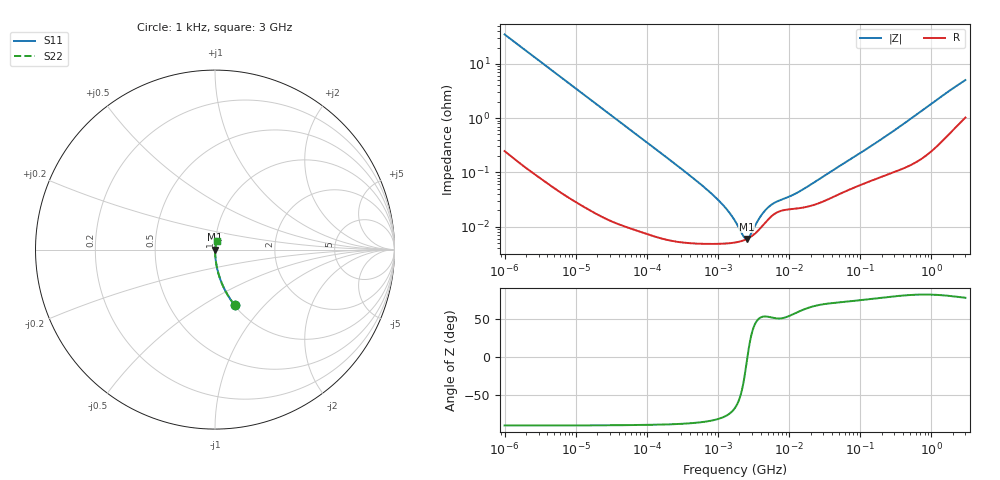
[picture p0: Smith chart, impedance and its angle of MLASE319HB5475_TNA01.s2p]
! MLASE319HB5475_TNA01  S-PARAMETER MODEL  ( Standard Model )
! Model Generated by TAIYO YUDEN Corporation (http://www.ty-top.com)
! Version 2.0
! TAIYO YUDEN Control No. 230906
! Copyright(c) 2009 TAIYO YUDEN CO.,LTD. All Rights Reserved.
! Product Description (link to TY-COMPAS)
! https://ds.yuden.co.jp/TYCOMPAS/or/detail?pn=MLASE319HB5475KTNA01&u=M
! Products Name : Multilayer Ceramic Capacitors
! Characteristics :
!  Capacitance : 4.7 [uF] , Rated Voltage : 16 [V] , TCC : B / X5R
!  Case Size : 3.2 x 1.6 / 0.126 x 0.063 [mm/inch] , Thickness : 0.85 / 0.033 [mm/inch]
!  (Conditions: Temperature = 25 [degC] , DC Bias Voltage = 0 [V])
! External Node Assignments :
!  1  o---| |---o  2
! GND o---------o GND
! Frequency Range : 1kHz  -  3GHz  [ 401 STEP ]
# MHZ S RI R 50
! Freq[MHz].  S11 Real  S11 Imag  S21 Real  S21 Imag  S12 Real  S12 Imag  S22 Real  S22 Imag
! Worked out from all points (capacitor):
!   401 points, 1 kHz to 3 GHz, reference 50 ohm
!   read as one part in series: C = 4.55 uF near 1.077 kHz
!   lowest |Z| = 5.9 mohm at 2.515 MHz (marker M1)
!   series resonance near 2.587 MHz, so ESL is about 830 pH
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0.001  0.1106 -0.3101  0.8894 0.3101  0.8894 0.3101  0.1106 -0.3101
0.001685  0.0427 -0.1987  0.9573 0.1987  0.9573 0.1987  0.0427 -0.1987
0.00306  0.0138 -0.1131  0.9862 0.1131  0.9862 0.1131  0.0138 -0.1131
0.005768  0.00415 -0.0608  0.9958 0.0608  0.9958 0.0608  0.00415 -0.0608
0.01216  0.00108 -0.029  0.9989 0.029  0.9989 0.029  0.00108 -0.029
0.147855  6.77e-05 -0.00241  0.9999 0.00241  0.9999 0.00241  6.77e-05 -0.00241
0.43594  4.95e-05 -0.000801  1 0.000801  1 0.000801  4.95e-05 -0.000801
0.821683  4.79e-05 -0.000395  1 0.000395  1 0.000395  4.79e-05 -0.000395
1.285341  4.86e-05 -0.000213  1 0.000213  1 0.000213  4.86e-05 -0.000213
1.732051  5.07e-05 -0.000117  0.9999 0.000117  0.9999 0.000117  5.07e-05 -0.000117
1.866149  5.16e-05 -9.43e-05  0.9999 9.43e-05  0.9999 9.43e-05  5.16e-05 -9.43e-05
2.010629  5.27e-05 -7.24e-05  0.9999 7.24e-05  0.9999 7.24e-05  5.27e-05 -7.24e-05
2.514714  5.84e-05 -8.04e-06  0.9999 8.04e-06  0.9999 8.04e-06  5.84e-05 -8.04e-06
3.03007  6.76e-05 4.55e-05  0.9999 -4.55e-05  0.9999 -4.55e-05  6.76e-05 4.55e-05
3.264662  7.31e-05 6.71e-05  0.9999 -6.71e-05  0.9999 -6.71e-05  7.31e-05 6.71e-05
4.566395  0.000116 0.000158  0.9999 -0.000158  0.9999 -0.000158  0.000116 0.000158
5.928204  0.000163 0.000208  0.9998 -0.000208  0.9998 -0.000208  0.000163 0.000208
12.03889  0.000213 0.000338  0.9998 -0.000338  0.9998 -0.000338  0.000213 0.000338
21.06097  0.000245 0.000567  0.9998 -0.000567  0.9998 -0.000567  0.000245 0.000567
256.0921  0.000961 0.00504  0.999 -0.00504  0.999 -0.00504  0.000961 0.00504
1714.862  0.00574 0.03  0.9943 -0.03  0.9943 -0.03  0.00574 0.03
3000  0.0125 0.0482  0.9875 -0.0482  0.9875 -0.0482  0.0125 0.0482
